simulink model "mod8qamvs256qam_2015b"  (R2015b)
settings: Solver=VariableStepAuto  SolverMode=SingleTasking  StartTime=0.0  StopTime=10  RelTol=1e-3
libraries: commdigbbndam3 x4, commchan3 x2, commsink2 x2, commrandsrc3 x2, dspsrcs4 x2

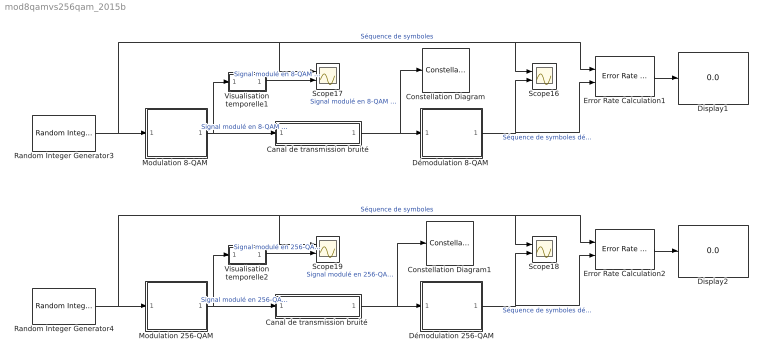
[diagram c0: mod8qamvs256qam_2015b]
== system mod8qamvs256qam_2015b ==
  Canal de transmission bruité : Subsystem
  "Canal de transmission bruité " : Subsystem
  Constellation Diagram : ConstellationDiagram
  Constellation Diagram1 : ConstellationDiagram
  Display1 : Display
  Display2 : Display
  Démodulation 256-QAM : Subsystem
  "Démodulation 8-QAM " : Subsystem
  Error Rate Calculation1 : commsink2/Error Rate Calculation  N=0  st_delay=0  cp_mode=Entire frame  subframe=[]  PMode=Port  WsName=ErrorVec  RsMode2=off  stop=off  numErr=100  maxBits=1e6
  Error Rate Calculation2 : commsink2/Error Rate Calculation  N=0  st_delay=0  cp_mode=Entire frame  subframe=[]  PMode=Port  WsName=ErrorVec  RsMode2=off  stop=off  numErr=100  maxBits=1e6
  Modulation 256-QAM : Subsystem
  "Modulation 8-QAM " : Subsystem
  Random Integer Generator3 : commrandsrc3/Random Integer Generator  SetSize=8  SeedSource=Auto  Seed=0  SampleTime=1  SamplesPerFrame=1  OutputDataType=double  SimulateUsing=Interpreted execution
  Random Integer Generator4 : commrandsrc3/Random Integer Generator  SetSize=256  SeedSource=Auto  Seed=0  SampleTime=1  SamplesPerFrame=1  OutputDataType=double  SimulateUsing=Interpreted execution
  Scope{16..19} (4 alike) : Scope  NumInputPorts=2
  Visualisation temporelle1 : Subsystem
  Visualisation temporelle2 : Subsystem
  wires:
  Random Integer Generator4/1 -> Modulation 256-QAM/1(In1), Error Rate Calculation2/1, Scope18/1, Scope19/1  "Séquence de symboles"
  "Canal de transmission bruité "/1(Out1) -> Constellation Diagram1/1, Démodulation 256-QAM/1(In1)  "Signal modulé en 256-QAM reçu"
  Error Rate Calculation2/1 -> Display2/1
  Modulation 256-QAM/1(Out1) -> "Canal de transmission bruité "/1(In1), Visualisation temporelle2/1(In1)  "Signal modulé en 256-QAM émis"
  Error Rate Calculation1/1 -> Display1/1
  Démodulation 256-QAM/1(Out1) -> Error Rate Calculation2/2, Scope18/2  "Séquence de symboles démodulé"
  "Démodulation 8-QAM "/1(Out1) -> Error Rate Calculation1/2, Scope16/2  "Séquence de symboles démodulé"
  "Modulation 8-QAM "/1(Out1) -> Canal de transmission bruité/1(In1), Visualisation temporelle1/1(In1)  "Signal modulé en 8-QAM émis"
  Canal de transmission bruité/1(Out1) -> Constellation Diagram/1, "Démodulation 8-QAM "/1(In1)  "Signal modulé en 8-QAM reçu"
  Visualisation temporelle2/1(Out1) -> Scope19/2  "Signal modulé en 256-QAM émis"
  Random Integer Generator3/1 -> "Modulation 8-QAM "/1(In1), Error Rate Calculation1/1, Scope16/1, Scope17/1  "Séquence de symboles"
  Visualisation temporelle1/1(Out1) -> Scope17/2  "Signal modulé en 8-QAM émis"

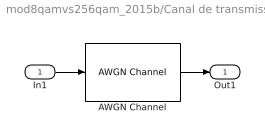
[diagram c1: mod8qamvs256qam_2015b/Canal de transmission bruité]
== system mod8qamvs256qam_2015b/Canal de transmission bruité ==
  In1 : Inport
  AWGN Channel : commchan3/AWGN Channel  InputProcessing=Columns as channels (frame based)  seed=67  noiseMode="Signal to noise ratio  (Eb/No)"  EbNodB=5  EsNodB=10  SNRdB=10  bitsPerSym=3  Ps=1  Tsym=1  variance=1
  Out1 : Outport
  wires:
  AWGN Channel/1 -> Out1/1
  In1/1 -> AWGN Channel/1

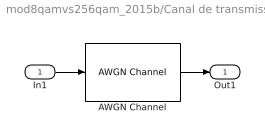
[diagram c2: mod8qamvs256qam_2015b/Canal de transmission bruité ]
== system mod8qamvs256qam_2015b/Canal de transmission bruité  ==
  In1 : Inport
  AWGN Channel : commchan3/AWGN Channel  InputProcessing=Columns as channels (frame based)  seed=67  noiseMode="Signal to noise ratio  (Eb/No)"  EbNodB=5  EsNodB=10  SNRdB=10  bitsPerSym=8  Ps=1  Tsym=1  variance=1
  Out1 : Outport
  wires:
  AWGN Channel/1 -> Out1/1
  In1/1 -> AWGN Channel/1

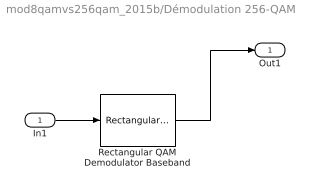
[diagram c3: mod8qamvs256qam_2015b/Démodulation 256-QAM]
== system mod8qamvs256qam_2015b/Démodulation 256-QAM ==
  In1 : Inport
  Rectangular QAM Demodulator Baseband : commdigbbndam3/Rectangular QAM Demodulator Baseband  M=256  OutType=Integer  DecType=Hard decision  VarSource=Dialog  Variance=1  Dec=Binary  Mapping=[0:15]  PowType=Min. distance between symbols  MinDist=0.5  AvgPow=1  PeakPow=1  Ph=0  outDtype1=Inherit via internal rule  outDtype2=Inherit via internal rule  derotateFactorWordLen=16  denormFactorWordLen=16  prodOutWordLen=32  prodOutOverflowMode=Wrap  prodOutRoundingMode=Floor  sumWordLen=32
  Out1 : Outport
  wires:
  Rectangular QAM Demodulator Baseband/1 -> Out1/1
  In1/1 -> Rectangular QAM Demodulator Baseband/1

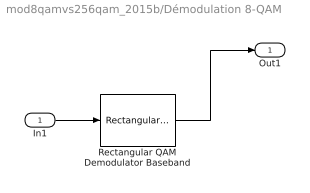
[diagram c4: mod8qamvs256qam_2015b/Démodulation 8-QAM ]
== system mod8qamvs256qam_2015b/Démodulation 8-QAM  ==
  In1 : Inport
  Rectangular QAM Demodulator Baseband : commdigbbndam3/Rectangular QAM Demodulator Baseband  M=8  OutType=Integer  DecType=Hard decision  VarSource=Dialog  Variance=1  Dec=Binary  Mapping=[0:15]  PowType=Min. distance between symbols  MinDist=2  AvgPow=1  PeakPow=1  Ph=0  outDtype1=Inherit via internal rule  outDtype2=Inherit via internal rule  derotateFactorWordLen=16  denormFactorWordLen=16  prodOutWordLen=32  prodOutOverflowMode=Wrap  prodOutRoundingMode=Floor  sumWordLen=32
  Out1 : Outport
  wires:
  Rectangular QAM Demodulator Baseband/1 -> Out1/1
  In1/1 -> Rectangular QAM Demodulator Baseband/1

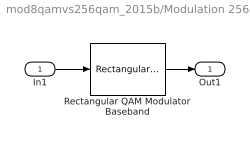
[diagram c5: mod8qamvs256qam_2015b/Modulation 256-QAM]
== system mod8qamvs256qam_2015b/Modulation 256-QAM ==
  In1 : Inport
  Rectangular QAM Modulator Baseband : commdigbbndam3/Rectangular QAM Modulator Baseband  M=256  InType=Integer  Enc=Binary  Mapping=[0:15]  PowType=Min. distance between symbols  MinDist=0.5  AvgPow=1  PeakPow=1  Ph=0  outDtype=double  outWordLen=16  outUDDataType=sfix(16)  outFracLenMode=Best precision  outFracLen=15
  Out1 : Outport
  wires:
  Rectangular QAM Modulator Baseband/1 -> Out1/1
  In1/1 -> Rectangular QAM Modulator Baseband/1

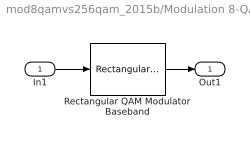
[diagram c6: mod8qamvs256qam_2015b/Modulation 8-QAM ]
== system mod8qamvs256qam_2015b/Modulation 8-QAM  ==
  In1 : Inport
  Rectangular QAM Modulator Baseband : commdigbbndam3/Rectangular QAM Modulator Baseband  M=8  InType=Integer  Enc=Binary  Mapping=[0:15]  PowType=Min. distance between symbols  MinDist=2  AvgPow=1  PeakPow=1  Ph=0  outDtype=double  outWordLen=16  outUDDataType=sfix(16)  outFracLenMode=Best precision  outFracLen=15
  Out1 : Outport
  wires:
  Rectangular QAM Modulator Baseband/1 -> Out1/1
  In1/1 -> Rectangular QAM Modulator Baseband/1

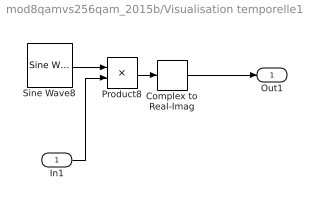
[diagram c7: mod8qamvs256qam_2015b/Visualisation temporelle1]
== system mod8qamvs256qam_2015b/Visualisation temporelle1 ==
  In1 : Inport
  Complex to Real-Imag : ComplexToRealImag  Output=Real
  Product8 : Product
  Sine Wave8 : dspsrcs4/Sine Wave  Amplitude=1  Frequency=1  Phase=0  SampleMode=Discrete  OutComplex=Complex  CompMethod=Trigonometric fcn  TableSize=Speed  SampleTime=1/100  SamplesPerFrame=1  ResetState=Restart at time zero  OutputFrames=off  dataType=double  wordLen=16  udDataType=sfix(16)  fracBitsMode=Best precision  numFracBits=15  OutDataTypeStr=double  LastOutDataTypeStr=double
  Out1 : Outport
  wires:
  Product8/1 -> Complex to Real-Imag/1
  Sine Wave8/1 -> Product8/1
  In1/1 -> Product8/2
  Complex to Real-Imag/1 -> Out1/1

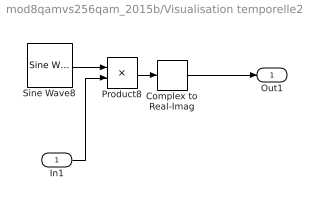
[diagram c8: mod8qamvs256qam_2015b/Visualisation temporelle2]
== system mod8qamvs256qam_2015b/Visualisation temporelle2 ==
  In1 : Inport
  Complex to Real-Imag : ComplexToRealImag  Output=Real
  Product8 : Product
  Sine Wave8 : dspsrcs4/Sine Wave  Amplitude=1  Frequency=1  Phase=0  SampleMode=Discrete  OutComplex=Complex  CompMethod=Trigonometric fcn  TableSize=Speed  SampleTime=1/100  SamplesPerFrame=1  ResetState=Restart at time zero  OutputFrames=off  dataType=double  wordLen=16  udDataType=sfix(16)  fracBitsMode=Best precision  numFracBits=15  OutDataTypeStr=double  LastOutDataTypeStr=double
  Out1 : Outport
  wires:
  Product8/1 -> Complex to Real-Imag/1
  Sine Wave8/1 -> Product8/1
  In1/1 -> Product8/2
  Complex to Real-Imag/1 -> Out1/1
